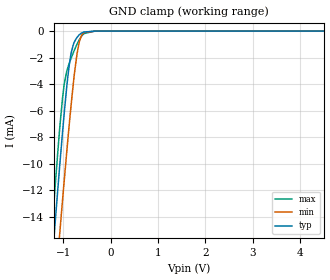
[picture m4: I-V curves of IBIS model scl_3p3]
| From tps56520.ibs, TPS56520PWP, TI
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|   scl_3p3 Model
[Model]   scl_3p3
Model_type   Input
Vinl = 0.6
Vinh = 1.8
|   typ   min   max
|   (nom PVT)   (fast PVT)   (slow PVT)
C_comp   6.933e-13   6.559e-13   7.326e-13
| Where nom  PVT is Nominal Process, 3.3V, 27C
|   Fast PVT is Strong Process,  3.6V, -40C
|   Slow PVT is Weak Process,   3V, 125C
[Voltage Range]   3.3   3   3.6
|Junction Temperature
[Temperature Range]   27   125   -40
[Power Clamp Reference]   3.3   3   3.6
[GND Clamp Reference]   0   0   0
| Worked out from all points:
|   GND clamp passes 1 mA (typ) near -0.79 V on its own axis
[GND Clamp]
|   Voltage   I(typ)   I(min)   I(max)
-3.3V     -117.9mA   -117.3mA   -124.6mA
-1.284V   -19.59mA   -24.35mA   -17.2mA
-1.231V   -17.14mA   -22.02mA   -14.57mA
-1.2V     -15.73mA   -20.66mA   -13.05mA
-1.162V   -13.98mA   -18.99mA   -11.21mA
-1.072V   -9.986mA   -15.11mA   -7.156mA
-974.4mV  -5.956mA   -11.03mA   -3.876mA
-858mV    -2.156mA   -6.43mA    -2.268mA
-785.4mV  -989.9uA   -3.864mA   -1.6mA
-711.6mV  -481.1uA   -1.751mA   -999.9uA
-596.4mV  -111.7uA   -217.6uA   -303.3uA
6.6V      0A         0A         0A
[POWER Clamp]
|   Voltage   I(typ)   I(min)   I(max)
-3.3V     0A         0A         0A
0V        0A         0A         0A
6.6V      0A         0A         0A
